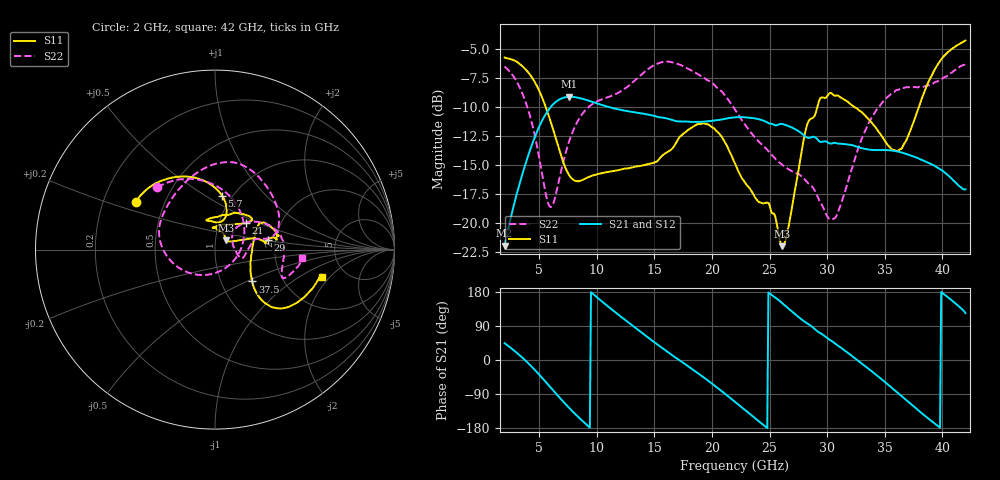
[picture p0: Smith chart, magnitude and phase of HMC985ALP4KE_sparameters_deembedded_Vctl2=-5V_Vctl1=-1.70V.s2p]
!s2p File: Measurements: S11, S21, S12, S22
# GHz S dB R 50.0
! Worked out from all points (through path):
!   401 points, 2 GHz to 42 GHz, reference 50 ohm
!   highest |S21| = -9.11 dB at 7.6 GHz (marker M1); lowest = -21.9 dB at 2 GHz (marker M2)
!   lowest |S11| = -22.0 dB at 26.1 GHz (marker M3), VSWR 1.17, Z = 56.2 + j5.81 ohm
!   |S11| at or under -10 dB: 5.574 GHz to 29.14 GHz (23.57 GHz wide, 136 % of centre); 32.37 GHz to 37.95 GHz (5.579 GHz wide, 15.9 % of centre)
!   |S22| runs from -19.7 to -6.1 dB; largest |S21 - S12| = 0.00043
!   S11 on the Smith chart (normalised r, x): 2 GHz: 0.34, +0.25; 5.7 GHz: 0.89, +0.59; 21 GHz: 1.34, +0.42; 29 GHz: 1.81, +0.22; 37.5 GHz: 1.40, -0.54; 42 GHz: 3.33, -1.61
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2  -5.73 148.8  -21.94 44.3  -21.95 44.2  -6.50 132.7
3.6  -6.53 122.5  -15.58 4.5  -15.58 4.5  -8.96 89.4
4.7  -7.98 101.5  -12.38 -28.6  -12.39 -28.6  -12.80 47.2
5.7  -10.35 82.7  -10.39 -62.4  -10.40 -62.4  -18.01 -21.5
6.2  -11.89 75.8  -9.77 -79.7  -9.77 -79.7  -18.36 -71.2
7.6  -15.86 76.9  -9.11 -126.3  -9.11 -126.3  -12.95 -153.2
8.7  -16.30 90.7  -9.26 -159.1  -9.27 -159.1  -10.64 178.0
12.1  -15.37 106.6  -10.24 114.3  -10.24 114.3  -8.62 131.3
15.4  -14.50 82.5  -10.86 37.9  -10.87 37.9  -6.20 83.6
18.1  -11.85 49.7  -11.26 -20.1  -11.26 -20.1  -6.78 52.6
21  -12.80 40.7  -11.02 -85.9  -11.03 -85.9  -8.82 16.9
22  -14.85 51.9  -10.87 -110.7  -10.88 -110.7  -10.21 12.1
24  -18.11 91.6  -11.02 -160.0  -11.03 -159.9  -12.89 14.2
26.1  -21.98 40.1  -11.45 150.0  -11.46 150.0  -14.96 -3.1
28.7  -10.96 7.2  -12.57 87.6  -12.57 87.6  -16.84 -16.5
29  -10.51 10.5  -12.62 79.6  -12.62 79.6  -17.32 -15.1
30.7  -9.02 14.5  -13.07 43.2  -13.08 43.2  -19.53 25.2
33.2  -10.62 30.2  -13.58 -13.9  -13.59 -13.9  -12.26 39.3
35.4  -13.40 7.8  -13.72 -68.0  -13.72 -67.9  -9.00 18.0
37.5  -11.28 -40.6  -14.24 -122.3  -14.25 -122.2  -8.29 -4.8
39.7  -6.17 -41.8  -15.27 -176.1  -15.27 -176.0  -7.71 -22.9
42  -4.25 -14.3  -17.07 123.8  -17.08 123.9  -6.25 -5.5
